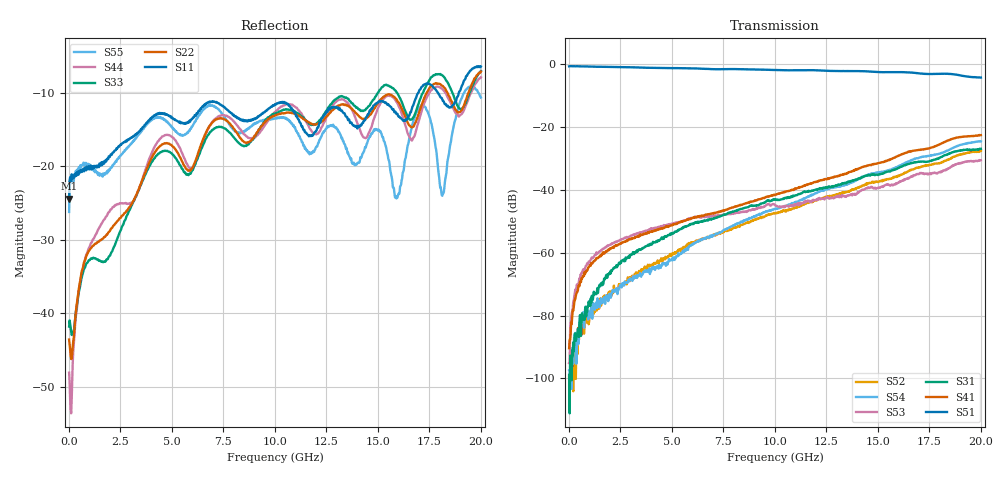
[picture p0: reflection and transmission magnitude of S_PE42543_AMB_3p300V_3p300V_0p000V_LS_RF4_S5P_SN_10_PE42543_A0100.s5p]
!Agilent Technologies,N5230C,MY49001593,A.09.33.09
!Agilent N5230C: A.09.33.09
!Date: Friday, March 21, 2014 07:24:10
!Correction: S11(Full 5 Port(1,2,3,5,6))
!S12(Full 5 Port(1,2,3,5,6))
!S13(Full 5 Port(1,2,3,5,6))
!S15(Full 5 Port(1,2,3,5,6))
!S16(Full 5 Port(1,2,3,5,6))
!S21(Full 5 Port(1,2,3,5,6))
!S22(Full 5 Port(1,2,3,5,6))
!S23(Full 5 Port(1,2,3,5,6))
!S25(Full 5 Port(1,2,3,5,6))
!S26(Full 5 Port(1,2,3,5,6))
!S31(Full 5 Port(1,2,3,5,6))
!S32(Full 5 Port(1,2,3,5,6))
!S33(Full 5 Port(1,2,3,5,6))
!S35(Full 5 Port(1,2,3,5,6))
!S36(Full 5 Port(1,2,3,5,6))
!S51(Full 5 Port(1,2,3,5,6))
!S52(Full 5 Port(1,2,3,5,6))
!S53(Full 5 Port(1,2,3,5,6))
!S55(Full 5 Port(1,2,3,5,6))
!S56(Full 5 Port(1,2,3,5,6))
!S61(Full 5 Port(1,2,3,5,6))
!S62(Full 5 Port(1,2,3,5,6))
!S63(Full 5 Port(1,2,3,5,6))
!S65(Full 5 Port(1,2,3,5,6))
!S66(Full 5 Port(1,2,3,5,6))
!S5P File: Measurements: <S11,S12,S13,S15,S16>,
!<S21,S22,S23,S25,S26>,
!<S31,S32,S33,S35,S36>,
!<S51,S52,S53,S55,S56>,
!<S61,S62,S63,S65,S66>:
# Hz S  dB  R 50
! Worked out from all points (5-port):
!   801 points, 10 MHz to 20 GHz, reference 50 ohm
!   strongest paths, dB at 10 MHz, 5.008 GHz, 10.01 GHz, 15 GHz, 20 GHz:
!     S51: -0.8, -1.4, -2.0, -2.6, -4.4
!     S41: -90.4, -51.3, -41.7, -31.6, -22.7
!     S31: -98.9, -53.8, -43.1, -35.4, -27.1
!     S53: -95.1, -50.8, -44.9, -39.5, -30.7
!     S54: -97.4, -61.9, -46.1, -34.5, -24.7
!     S52: -99.7, -60.4, -47.5, -37.6, -27.7
!   lowest |S11| = -24.5 dB at 10 MHz (marker M1), VSWR 1.13, Z = 56 - j2.1 ohm
!   |S11| at or under -10 dB: start of sweep to 16.97 GHz; 17.9 GHz to 18.93 GHz (1.029 GHz wide, 5.59 % of centre)
